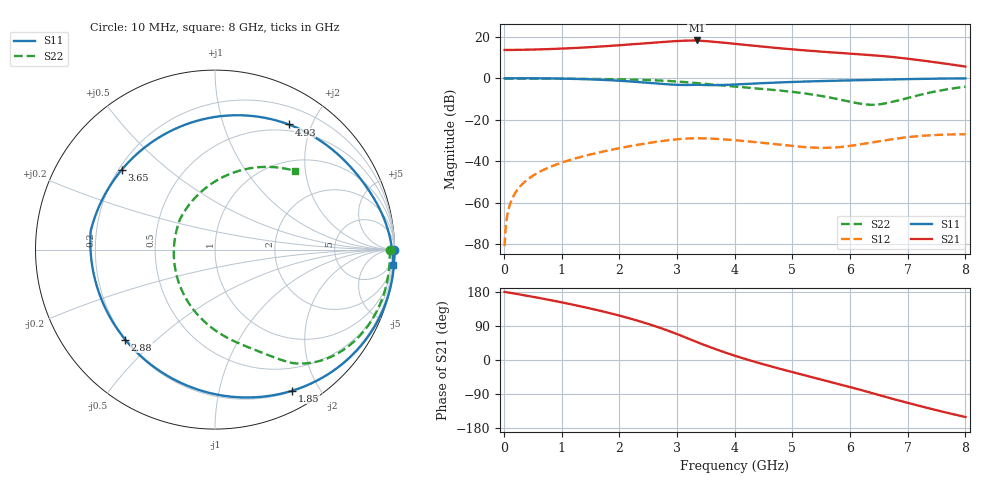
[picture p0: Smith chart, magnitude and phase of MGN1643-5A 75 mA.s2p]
! Port[1] = GATE
! Port[2] = DRAIN
! [Type]  S-parameter s2p file touchstone ver. 1.0
! [Object]  MGN1643-5A
! [Bias]  75 mA
! [Version]  1.0
! [Date]  Thu May 19 10:52:50 2026
! [Source]  This file was created in JSC "ICC Milandr".
! [Disclaimer] Property of JSC "ICC Milandr". Unauthorized reproduction and/or distribution is strictly prohibited.
!  The file and the data are provided "AS IS" and with all faults and disclaim all warranties, express and implied, including
!  without limitation any implied warranties of merchantability, fitness for a particular purpose.
!  JSC "ICC Milandr" assumes no liability for:
!  1) the accuracy of the data provided;
!  2) the proper functioning of this data;
!  3) infringement of patents, copyrights or intellectual property rights resulting from the use of this data.
!  JSC "ICC Milandr" reserves the right to make changes to the products and the data without prior notice.
!  Please, be aware that your receipt and use of the file provided shall serve as acceptance of these terms and conditions.
!  If you do not accept these terms, you should return or destroy this file and any other accompanying information immediately.
# Hz S MA R 12.5
! freq  S11mag  S11ang  S21mag  S21ang  S12mag  S12ang  S22mag  S22ang
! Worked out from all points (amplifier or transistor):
!   800 points, 10 MHz to 8 GHz, reference 12.5 ohm
!   highest |S21| = 18.3 dB at 3.34 GHz (marker M1)
!   |S21| within 3 dB of that: 1.637 GHz to 4.493 GHz (2.855 GHz wide, 93.2 % of centre)
!   unconditionally stable (mu >= 1): 4.981 GHz to 5.668 GHz
!   at 1.34 GHz: K = 0.23, MSG = 26.3 dB, |S12| = -37.9 dB
!   at 4.01 GHz: K = 0.72, MSG = 23.3 dB, |S12| = -29.9 dB
!   at 8 GHz: K = 0.25, MSG = 16.3 dB, |S12| = -27.0 dB
!   S11 on the Smith chart (normalised r, x): 10 MHz: open; 1.85 GHz: 0.21, -1.67; 2.88 GHz: 0.20, -0.40; 3.65 GHz: 0.21, +0.36; 4.93 GHz: 0.41, +1.67; 8 GHz: 1, -23
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1e7  1 -0.2  4.832 179.7  8.859e-05 86.4  0.973 -0.1
1.1e8  1.001 -3.0  4.836 177.2  0.0009655 87.4  0.9738 -1.4
3.1e8  1.001 -8.4  4.871 172.0  0.002734 83.6  0.9751 -4.1
8.9e8  0.9879 -25.2  5.128 155.5  0.008119 71.1  0.9747 -12.0
1.35e9  0.9571 -40.6  5.49 140.9  0.01285 59.7  0.9681 -18.7
1.85e9  0.8965 -61.2  6.06 123.0  0.01866 45.5  0.9516 -26.6
2.28e9  0.8209 -84.9  6.712 105.4  0.0243 31.0  0.9256 -34.1
2.68e9  0.7412 -115.4  7.413 86.2  0.02979 14.6  0.885 -42.0
2.88e9  0.7084 -134.9  7.747 75.4  0.03231 5.1  0.8561 -46.2
3.11e9  0.6894 -160.7  8.046 61.9  0.0346 -6.8  0.8147 -51.0
3.34e9  0.7002 171.4  8.183 47.5  0.03579 -19.7  0.7663 -55.6
3.49e9  0.6869 155.4  7.914 38.7  0.03539 -26.9  0.7322 -58.0
3.65e9  0.6841 139.3  7.583 29.6  0.03461 -34.0  0.6982 -60.3
3.82e9  0.6916 123.8  7.205 20.5  0.03347 -40.8  0.665 -62.7
4.01e9  0.7081 108.5  6.779 10.9  0.03194 -47.2  0.631 -65.5
4.45e9  0.7584 80.8  5.872 -9.3  0.02793 -57.2  0.5601 -73.0
4.93e9  0.8092 59.5  5.085 -29.1  0.0237 -59.6  0.4821 -84.3
5.34e9  0.8441 46.0  4.568 -45.2  0.02125 -53.4  0.4065 -98.2
6.02e9  0.8914 29.1  3.913 -72.1  0.02354 -33.9  0.2679 -140.2
6.67e9  0.9358 16.4  3.342 -99.8  0.03277 -27.9  0.2592 138.2
7.3e9  0.9709 6.1  2.631 -124.9  0.0413 -44.5  0.4248 79.9
8e9  0.9955 -5.0  1.917 -150.4  0.04462 -64.0  0.6262 44.4
